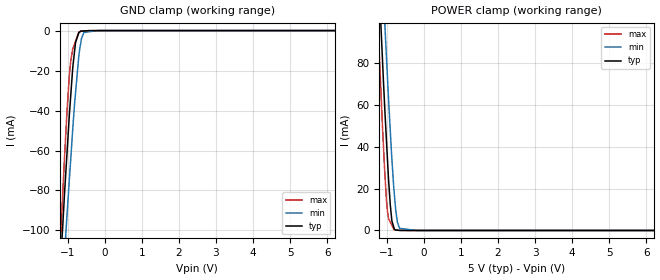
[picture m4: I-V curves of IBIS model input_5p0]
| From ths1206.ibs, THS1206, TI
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|   input_5p0 Model
[Model]   input_5p0
Model_type   Input
Vinl = 0.6
Vinh = 2.6
|   typ   min   max
|   (nom PVT)   (fast PVT)   (slow PVT)
C_comp   9.597e-13   9.486e-13   9.672e-13
| Where nom  PVT is Nominal Process, 5V, 43C
|   Fast PVT is Strong Process,  5.25V, -55C
|   Slow PVT is Weak Process,   4.75V, 145C
[Voltage Range]   5   4.75   5.25
|Ambient Temperature   25   125   -55
|Junction Temperature
[Temperature Range]   43   145   -55
[Power Clamp Reference]   5   4.75   5.25
[GND Clamp Reference]   0   0   0
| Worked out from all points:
|   GND clamp passes 1 mA (typ) near -0.69 V on its own axis
|   POWER clamp passes 1 mA (typ) near -0.80 V on its own axis
[GND Clamp]
|   Voltage   I(typ)   I(min)   I(max)
-5V       -1.63A     -1.558A    -1.765A
-1.306V   -156.5mA   -182mA     -149mA
-1.08V    -80.95mA   -111.4mA   -62.58mA
-1.021V   -63.13mA   -93.97mA   -42.58mA
-913.5mV  -32.25mA   -64mA      -15.06mA
-855mV    -17.62mA   -47.73mA   -8.966mA
-785mV    -5.956mA   -31.17mA   -5.31mA
-698.3mV  -1.195mA   -13.09mA   -779.1uA
-640.5mV  -317.8uA   -5.762mA   -155.4uA
-560.5mV  -201.6uA   -951.6uA   -136uA
-190mV    0A         -86.58nA   -46.1uA
10V       0A         0A         0A
[POWER Clamp]
|   Voltage   I(typ)   I(min)   I(max)
-5V       1.779A     1.789A     1.781A
-1.306V   156.4mA    196.8mA    126.8mA
-1.118V   82.82mA    123.8mA    50.84mA
-1.045V   55.24mA    96.12mA    25.4mA
-981.8mV  34.27mA    73.56mA    9.276mA
-905mV    12.27mA    47.74mA    4.047mA
-860mV    4.468mA    33.7mA     2.404mA
-803.3mV  1.116mA    18.99mA    330.8uA
-712.5mV  144.4uA    4.022mA    160.9uA
-655.5mV  45.75uA    1.019mA    54.14uA
-190mV    0A         0A         7.728uA
10V       0A         0A         0A
